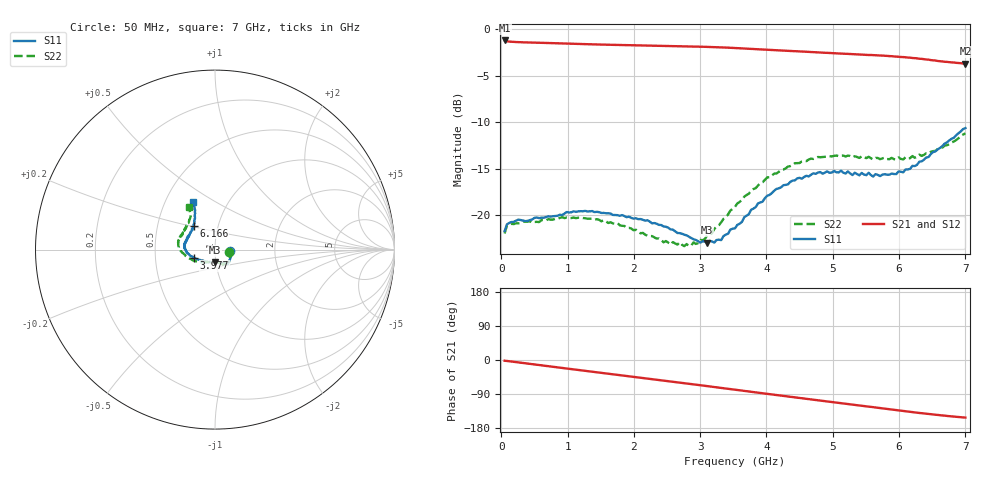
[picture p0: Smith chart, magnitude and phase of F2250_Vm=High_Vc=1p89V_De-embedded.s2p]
! Integrated Device Technology
! Corporate Headquarters
! 6024 Silver Creek Valley Road
! San Jose, CA 95138  USA
! Phone:  1-408-284-8200
! Toll Free:  1-800-223-1366
! Webpage:  http://www.idt.com/
! Timing and RF Division
! 515 Groton Road, Suite 102
! Westford, MA 01886-6024
! Device:  F2250
! Description: Voltage Variable RF Attenuator
! Frequency:  50.0 -  6000.00 MHz
! Package:  3x3 mm Thin QFN Plastic Package: 16 pin
! Ports:  2 RF, 3 DC
!  Pin  1  = GND
!  Pin  2  = NC
!  Pin  3  = RF1  = Port 1
!  Pin  4  = NC
!  Pin  5  = GND
!  Pin  6  = GND
!  Pin  7  = GND
!  Pin  8  = GND
!  Pin  9  = NC
!  Pin 10  = RF2  = Port 2
!  Pin 11  = NC
!  Pin 12  = GND
!  Pin 13  = GND
!  Pin 14  = VCNTRL
!  Pin 15  = VDD
!  Pin 16  = VMODE
! Vcntrl:  1.890 Volts
! Vmode:  +3.300 Volts
! Vdd:  +3.30  Volts
! Current:  1.321 mA
! Data:  The device was measured on a the F2250 evaluation board which has
!  individual transmission lines to the RF pins.  Data was collected
!  using a calibrated network analyzer.  The evaluation board was
!  de-embedded using a TRL calibration technique.
!  The reference plane is the edge of the package pin.
! Misc:  SN 10
!  Action Tracker AT0258
! Date Measured:  2014-11-26
! Date:  2015-10-15  MJV
! Note:
!  Integrated Device Technology supplies this data as a sample of measured
!  data at the package pin for this product.  Your particular data for this
!  product may vary.
!  Data was taken at 25 degrees C.
!  Integrated Device Technology reserves the right to change this data at anytime.
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# GHz S dB R 50
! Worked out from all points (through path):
!   201 points, 50 MHz to 7 GHz, reference 50 ohm
!   highest |S21| = -1.19 dB at 50 MHz (marker M1); lowest = -3.7 dB at 7 GHz (marker M2)
!   group delay of S21, straight-line fit = 61.1 ps
!   lowest |S11| = -22.9 dB at 3.108 GHz (marker M3), VSWR 1.15, Z = 49.2 - j7.06 ohm
!   |S11| at or under -10 dB: start of sweep to end of sweep
!   |S22| runs from -23.3 to -11.2 dB; largest |S21 - S12| = 0.0018
!   S11 on the Smith chart (normalised r, x): 50 MHz: 1.18, -0.02; 3.977 GHz: 0.79, -0.07; 6.166 GHz: 0.76, +0.21; 7 GHz: 0.68, +0.40
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0.05  -21.70 -6.8  -1.19 -1.8  -1.19 -1.8  -21.94 -7.8
0.08475  -20.96 -6.5  -1.27 -2.5  -1.27 -2.5  -21.11 -7.2
0.1195  -20.81 -7.1  -1.31 -3.3  -1.31 -3.3  -20.94 -7.1
0.71025  -20.09 -30.6  -1.46 -16.4  -1.46 -16.5  -20.40 -34.0
1.2315  -19.55 -46.3  -1.58 -27.9  -1.58 -27.9  -20.28 -54.2
1.75275  -19.97 -53.3  -1.67 -39.1  -1.67 -39.1  -20.83 -63.6
2.37825  -21.02 -55.4  -1.76 -52.7  -1.76 -52.7  -22.47 -71.3
2.552  -21.50 -59.1  -1.78 -56.5  -1.78 -56.5  -23.13 -77.7
2.691  -21.90 -64.5  -1.80 -59.6  -1.80 -59.6  -22.90 -84.1
2.83  -22.29 -69.9  -1.82 -62.7  -1.82 -62.7  -23.28 -92.8
3.108  -22.93 -92.0  -1.88 -69.0  -1.88 -69.0  -22.13 -115.1
3.3165  -22.65 -112.5  -1.93 -73.7  -1.93 -73.8  -20.73 -129.9
3.4555  -21.51 -126.0  -1.97 -76.9  -1.97 -76.9  -19.47 -138.4
3.525  -21.39 -130.7  -2.00 -78.4  -2.00 -78.5  -19.07 -141.9
3.97675  -18.13 -158.5  -2.17 -88.6  -2.16 -88.6  -16.17 -162.8
4.4285  -16.23 -173.1  -2.34 -98.6  -2.35 -98.6  -14.39 -177.3
4.7065  -15.47 178.9  -2.44 -104.7  -2.45 -104.7  -13.93 176.4
5.054  -15.36 170.4  -2.57 -112.4  -2.57 -112.4  -13.56 168.8
5.85325  -15.61 143.5  -2.87 -129.8  -2.87 -130.0  -13.95 149.3
6.166  -15.00 131.5  -3.04 -136.7  -3.04 -136.8  -13.84 140.7
6.54825  -13.11 120.9  -3.34 -144.6  -3.34 -144.7  -13.05 128.5
7  -10.61 115.0  -3.67 -152.0  -3.68 -152.1  -11.18 121.9
